(* Logix 5000 AddOnInstructionDefinition export MPLS_Yaskawa; software revision 17.00 *)

TYPE Yaskawa_PLS_Switch :   // Structure of parameters needed for PLS switch operation using MPLS_Yaskawa v2.4.0
STRUCT
   FlagNumber : INT;   // Assigns a Flag number to the PLS output channel. Must be a physical output Flag 73-80, 88-90.
   OnPosition : REAL;   // If OnPosition < OffPosition output is ON between them. If OnPosition > OffPosition output is OFF between them and ON everywhere else.
   OffPosition : REAL;
   OnCompensation : INT;   // [msec]. Negative number turns output on SOONER, positive number turns output on LATER.
   OffCompensation : INT;   // [msec]
END_STRUCT
END_TYPE

TYPE Yaskawa_EIP_Servo :   // Yaskawa SigmaLogic Axis Structure v2.4.0
STRUCT
   O : Yaskawa_OUT_to_Servo;
   I : Yaskawa_IN_from_Servo;
   AOI_SB : Yaskawa_AOI_Status_Bits;
END_STRUCT
END_TYPE

TYPE Yaskawa_OUT_to_Servo :   // Structure of data sent out to the Yaskawa SigmaLogic controller v2.4.0
STRUCT
   b00_ServoOn : BOOL;   // Servo On
   b01_Stop : BOOL;   // Stops All Current Motion in Progress
   b02_Home : BOOL;   // Start Homing Process
   b03_MoveStart1 : BOOL;   // Start Current Motion
   b06_SuperImpose : BOOL;
   b07_ServoAlarmReset : BOOL;   // Servo Alarm Reset
   b08_ControllerAlarmReset : BOOL;   // SigmaLogic Alarm Reset
   b09_MoveStart2 : BOOL;   // Start Second Motion (Blended Move)
   b10_MoveAbort : BOOL;   // Abort Current Move
   b11_MovePause : BOOL;   // Pause Current Move
   b12_SeqPause : BOOL;   // Indexing Sequence Pause
   b13_SeqResume : BOOL;   // Indexing Sequence Resume
   b14_SeqCancel : BOOL;   // Indexing Sequence Cancel
   b15_AbsEncoderReset : BOOL;   // Absolute Encoder Reset
   b16_SeqStart : BOOL;   // Start Indexing Sequence
   b17_SeqEditSpeed : BOOL;   // Enter Edit Speed
   b18_SeqEditDistance : BOOL;   // Enter Distance Edit
   b19_PLSEnable : BOOL;   // Enable PLS execution
   b20_PLSActivateOutput1 : BOOL;   // Activate PLS output1 switch logic
   b21_PLSActivateOutput2 : BOOL;   // Activate PLS output2 switch logic
   b22_PLSActivateOutput3 : BOOL;   // Activate PLS output3 switch logic
   b23_PLSActivateOutput4 : BOOL;   // Activate PLS output4 switch logic
   b24_SetClock : BOOL;   // Set the remote controller clock with data provided by the PLC
   RebootController : BOOL;
   UseExternalEncoder : BOOL;   // Use External Encoder when executing MAHSP_Yaskawa
   b32_HeatbeatAnswer : BOOL;   // Heartbeat Answer
   BrakeBypassRequest : BOOL;
   SetFwdTorqueLimit : BOOL;
   SetRevTorqueLimit : BOOL;
   TorqueLimit : DINT;
   TorqueRamp : DINT;
   HomeMethod : INT;
   HomeSpeed : DINT;
   HomeAccDec : DINT;   // Home Move Acceleration/Deceleration Rate
   HomeBackOffDistance : DINT;
   HomeCreepSpeed : DINT;
   HomeCreepDistanceLimit : DINT;
   HomeCreepTimeLimit : DINT;
   HomeOffsetDistance : DINT;
   HomeOffsetSpeed : DINT;
   HomePostion : DINT;
   HomeTorque : DINT;
   HomeInputNo : DINT;
   HomeApproachTimeLimit : DINT;
   HomeApproachDistLimit : DINT;
   HomeDirection : INT;
   HomeSwitchMode : INT;
   MoveType : INT;
   MoveDirection : INT;
   MoveAccel1 : DINT;
   MoveAccel2 : DINT;
   MoveDecel1 : DINT;
   MoveDecel2 : DINT;
   MoveSpeed1 : DINT;
   MoveSpeed2 : DINT;
   MoveDistance1 : DINT;
   MoveDistance2 : DINT;
   MovePosition1 : DINT;
   MovePosition2 : DINT;
   RegistrationDistance : DINT;
   GearNumerator : DINT;
   GearDenominator : DINT;
   SuperImposeDistance : DINT;
   Resolution : INT;
   RegistrationDirection : INT;
   TuningLevel : INT;
   SequenceStep : INT;   // Staring Sequence Step Number
   SequenceEditStep : INT;   // Sequence Step Number to Edit
   FlagCommandBits1 : DINT;   // Flag Commands. 1..64 are General Flags, Bits 0..31 correspond to Flag 1..32
   FlagCommandBits2 : DINT;   // Flag Commands cont. 1..64 are General Flags, Bits 0..31 correspond to Flag 33..64
   DigitalOutCommandBits : DINT;   // Digital Output commands. Bits 0-7 correspond to CN13 Digital Outputs 0-7, used as Flag 73-80. Bits 8-10 correspond to CN1 Digital Outputs 0-2 used as Flag 88-90"
   SequenceEditSpeed : DINT;
   SequenceEditDistance : DINT;
   FeedRateOverride : INT;
   HSI_Enable : BOOL;
   HSI_MoveMode : BOOL;   // 0=Relative; 1=Moves per Cycle
   HSI_CalcMethod : BOOL;   // 0=Accel/Decel; 1=Time
   HSI_MoveDirection : BOOL;   // 0 = Negative; 1 = Positive
   HSI_TriggerFlag : INT;
   HSI_MovingFlag : INT;
   HSI_DwellingFlag : INT;
   HSI_DoneFlag : INT;
   HSI_MoveType : INT;   // 0=Single; 1=Repeat; 2=Repeat "x" times
   HSI_RepeatNumber : INT;
   HSI_Distance : DINT;
   HSI_Speed : DINT;
   HSI_Accel : DINT;
   HSI_MoveTime : DINT;
   HSI_DwellTime : DINT;
   PLS_OutputFlag1 : INT;
   PLS_OutputFlag2 : INT;
   PLS_OutputFlag3 : INT;
   PLS_OutputFlag4 : INT;
   PLS_OnPosition1 : DINT;
   PLS_OffPosition1 : DINT;
   PLS_OnPosition2 : DINT;
   PLS_OffPosition2 : DINT;
   PLS_OnPosition3 : DINT;
   PLS_OffPosition3 : DINT;
   PLS_OnPosition4 : DINT;
   PLS_OffPosition4 : DINT;
   PLS_OnCompensation1 : INT;
   PLS_OffCompensation1 : INT;
   PLS_OnCompensation2 : INT;
   PLS_OffCompensation2 : INT;
   PLS_OnCompensation3 : INT;
   PLS_OffCompensation3 : INT;
   PLS_OnCompensation4 : INT;
   PLS_OffCompensation4 : INT;
   RTC_Year : INT;
   RTC_Month : INT;
   RTC_Day : INT;
   RTC_Hour : INT;
   RTC_Min : INT;
   RTC_Sec : INT;
   StopDecel : DINT;
   AnalogOutput : INT;   // CN13, AO_01 [mV]
END_STRUCT
END_TYPE

TYPE Yaskawa_AOI_Status_Bits :   // Internal bits used to interlock Yaskawa AOI execution. v2.4.0
STRUCT
   MAM : BOOL;   // Move AOI Active
   MAJ : BOOL;   // Jog AOI Active
   MAB : BOOL;   // Blending AOI Active
   MAG : BOOL;   // Gearing AOI Active
   MAHSP : BOOL;   // Home SetPoint AOI Active
   MAH : BOOL;   // Homing AOI Active
   MSQE : BOOL;   // Sequence Edit AOI Active
   MSQR : BOOL;   // Sequence Run AOI Active
   MHSI : BOOL;   // High Speed Index AOI Active
   MSO : BOOL;   // Servo On
   MSF : BOOL;   // Servo Off
   MAFR : BOOL;   // Fault Reset
   MAS : BOOL;   // Servo Abort
   MTRQ : BOOL;   // Torque Mode Active
   MPLS : BOOL;   // PLS Active
   MCLK : BOOL;   // SetClock Active
   MSTL : BOOL;   // Set Torque Limit Active
   AOI_Permissive : BOOL;   // Permissive to Execute an AOI
END_STRUCT
END_TYPE

TYPE Yaskawa_IN_from_Servo :   // Structure of data coming from the Yaskawa SigmaLogic controller. v2.4.0
STRUCT
   AlarmText : STRING;   // ServoPack Alarm Code plus Text Description
   b00_Heartbeat : BOOL;
   b01_Alarm : BOOL;   // ServoPack Alarm
   b02_Warning : BOOL;   // ServoPack Warning
   b03_Ready : BOOL;   // ServoPack Ready
   b04_Enabled : BOOL;   // ServoPack Enabled ("Servo On")
   b05_StopComplete : BOOL;
   b06_HomeComplete : BOOL;
   b07_HomeBusy : BOOL;
   b08_HomeActive : BOOL;
   b09_HomeAborted : BOOL;
   b10_HomeError : BOOL;
   b11_MoveAbsComplete : BOOL;
   b12_MoveAbsBusy : BOOL;
   b13_MoveAbsActive : BOOL;
   b14_MoveAbsAborted : BOOL;
   b15_MoveAbsError : BOOL;
   b16_MoveRelComplete : BOOL;
   b17_MoveRelBusy : BOOL;
   b18_MoveRelActive : BOOL;
   b19_MoveRelAborted : BOOL;
   b20_MoveRelError : BOOL;
   b21_JogAtSpeed : BOOL;
   b22_JogBusy : BOOL;
   b23_JogActive : BOOL;
   b24_JogAborted : BOOL;
   b25_JogError : BOOL;
   b26_GearInSync : BOOL;
   b27_GearBusy : BOOL;
   b28_GearActive : BOOL;
   b29_GearAborted : BOOL;
   b30_GearError : BOOL;
   b32_MoveSuperComplete : BOOL;
   b33_MoveSuperBusy : BOOL;
   b34_MoveSuperActive : BOOL;
   b35_MoveSuperAborted : BOOL;
   b36_MoveSuperError : BOOL;
   b37_PowerCycleRequired : BOOL;
   b38_MoveBlend1Complete : BOOL;
   b39_MoveBlend1Busy : BOOL;
   b40_MoveBlend1Active : BOOL;
   b41_MoveBlend1Abort : BOOL;
   b42_MoveBlend1Error : BOOL;
   b43_MoveBlend2Complete : BOOL;
   b44_MoveBlend2Busy : BOOL;
   b45_MoveBlend2Active : BOOL;
   b46_MoveBlend2Abort : BOOL;
   b47_MoveBlend2Error : BOOL;
   b48_RegComplete : BOOL;
   b49_RegBusy : BOOL;
   b50_RegActive : BOOL;
   b51_RegAborted : BOOL;
   b52_RegError : BOOL;
   b53_ResetAbsEncoderActive : BOOL;
   b54_ResetAbsEncoderBusy : BOOL;
   b55_ResetAbsEncoderDone : BOOL;
   b56_ResetAbsEncoderError : BOOL;
   b57_SeqRunning : BOOL;
   b58_RegSensorNotReached : BOOL;
   b59_SeqEditError : BOOL;
   b60_SeqEditDone : BOOL;
   b61_TorqueAtTorque : BOOL;
   b62_TorqueBusy : BOOL;
   b63_TorqueActive : BOOL;
   b64_TorqueAborted : BOOL;
   b65_TorqueError : BOOL;
   b66_ControllerAlarm : BOOL;
   b67_ApplicationError : BOOL;
   b68_AxisAtStandStill : BOOL;
   b69_TestModeActive : BOOL;
   b70_ServoParamsOK : BOOL;
   b71_SetFwdTorqueLimitDone : BOOL;
   b72_SetRevTorqueLimitDone : BOOL;
   Position : DINT;
   Speed : DINT;
   Torque : DINT;
   HomeErrorID : INT;
   MoveAbsErrorID : INT;
   MoveRelErrorID : INT;
   JogErrorID : INT;
   GearErrorID : INT;
   MoveSuperErrorID : INT;
   ServoAlarmID : INT;
   ServoWarningID : INT;
   ControllerAlarmID : DINT;
   AxisGenAlarmID : DINT;
   MoveBlend1ErrorID : INT;
   MoveBlend2ErrorID : INT;
   ResetAbsEncoderErrorID : INT;
   FunctionBlockErrorID : INT;
   TorqueErrorID : INT;
   RegErrorID : INT;
   SeqCurrentStep : INT;
   FlagStatusBit1 : DINT;   // Flag Status. 1..64 are General Flags, Bits 0..31 correspond to Flag 1..32
   FlagStatusBit2 : DINT;   // Flag Status cont. 1..64 are General Flags, Bits 0..31 correspond to Flag 33..64
   IOStatusBits : DINT;   // Digital IO Status. Bits 0-7, CN13 Inputs 0-7, Used as Flag 65-72. Bits 8-15, CN13 Outputs 0-7, Used as Flag 73-80. Bits 16-22, CN1 Inputs 0-6, Used as Flag 81-87. Bits 23-25, CN1 Outputs 0-4, Used as Flag 88-92.
   HSI_Moving : BOOL;
   HSI_Dwelling : BOOL;
   HSI_Done : BOOL;
   HSI_Busy : BOOL;
   HSI_Error : BOOL;
   HSI_ErrorCode : INT;
   PLS_Running : BOOL;
   PLS_SwitchStatus1 : BOOL;
   PLS_SwitchStatus2 : BOOL;
   PLS_SwitchStatus3 : BOOL;
   PLS_SwitchStatus4 : BOOL;
   PLS_Busy : BOOL;
   PLS_Error : BOOL;
   PLS_ErrorCode : INT;
   SetClock_Done : BOOL;
   SetClock_Busy : BOOL;
   SetClock_Error : BOOL;
   SetClock_ErrorID : INT;
   SoftwareVersion : DINT;
   FirmwareVersion : DINT;
   CommandedPos : DINT;
   CommandedPosNonCyc : DINT;
   CommandedSpeed : DINT;
   Clock_Year : INT;
   Clock_Month : INT;
   Clock_Day : INT;
   Clock_Hour : INT;
   Clock_Minute : INT;
   Clock_Second : INT;
   AnalogInput : REAL;   // CN13, AI_01 [v]
   BrakeBypassActive : BOOL;
   ForwardTorqueLimit : DINT;
   ReverseTorqueLimit : DINT;
END_STRUCT
END_TYPE

ADD_ON_INSTRUCTION MPLS_Yaskawa   (* revision 2.4 0, vendor Yaskawa America, Inc., ExecuteEnableInFalse *)
// Motion Programmable Limit Switch
// Revision note:
// 2.4.0: No functional change
// 2.3.1: No functional change
// 2.3.0: No functional change
// 2.0.0: Improved output operation and error code reporting. Improved interlocking with embedded code.
// 1.2.0: No functional change.
// Initial Release 9/10/2014
// Help:
// This AOI transfers settings to the remote axis node for high-response of local outputs in relation to servo position. This block can run simultaneously with other motion function blocks. Up to four local digital outputs can be configured as a PLS output. Each has a single switch for OnPosition and OffPosition in relation to the servo axis position. Automatic Speed Compensation is supported independently for the OnPosition and for the OffPosition. Output Time Duration limiting is NOT supported at this time. However, the main PLC can easily monitor the switch output signals and deactivate the switch from the application code if a certain time limit is exceeded.
// SwitchData is a structure consisting of:
// - FlagNumber [INT]
// - OnPosition [REAL]
// - OffPosition [REAL]
// - OnCompensation [INT]
// - OffCompensation [INT]
VAR_IN_OUT
   Axis : Yaskawa_EIP_Servo; {required}
END_VAR
VAR_OUTPUT
   EN : BOOL; {visible}   // AOI is Active
   DN : BOOL; {visible}   // PLS_Busy
   IP : BOOL; {visible}   // PLS_Running
   ER : BOOL; {visible}   // PLS_Error
END_VAR
VAR_IN_OUT
   Switch1Data : Yaskawa_PLS_Switch; {required}
   Switch2Data : Yaskawa_PLS_Switch; {required}
   Switch3Data : Yaskawa_PLS_Switch; {required}
   Switch4Data : Yaskawa_PLS_Switch; {required}
END_VAR
VAR_INPUT
   ActivateSwitch1 : BOOL; {required}
   ActivateSwitch2 : BOOL; {required}
   ActivateSwitch3 : BOOL; {required}
   ActivateSwitch4 : BOOL; {required}
END_VAR
VAR_OUTPUT
   S1 : BOOL; {visible}   // Switch1 Status
   S2 : BOOL; {visible}   // Switch2 Status
   S3 : BOOL; {visible}   // Switch3 Status
   S4 : BOOL; {visible}   // Switch4 Status
   FLT_RDY : BOOL; {visible}   // The Servo is Not Ready
   FLT_BSY : BOOL;   // There is another AOI Active for this Axis
   ErrorCode : DINT; {visible}   // Fault code for PLS function
END_VAR
VAR
   AOI_ON_LOCAL : BOOL;
   ScaleFactor : DINT;
END_VAR

ROUTINE EnableInFalse   (* ladder *)
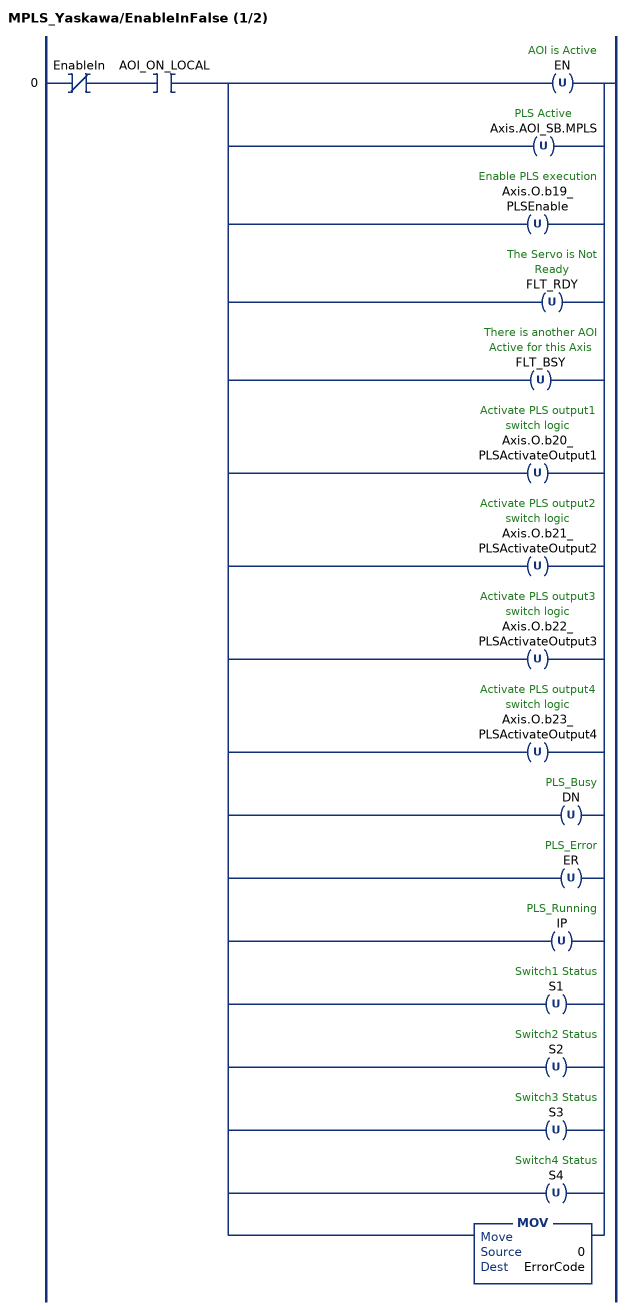
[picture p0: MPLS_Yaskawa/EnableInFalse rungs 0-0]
   0: XIO(EnableIn)XIC(AOI_ON_LOCAL)[OTU(EN) ,OTU(Axis.AOI_SB.MPLS) ,OTU(Axis.O.b19_PLSEnable) ,OTU(FLT_RDY) ,OTU(FLT_BSY) ,OTU(Axis.O.b20_PLSActivateOutput1) ,OTU(Axis.O.b21_PLSActivateOutput2) ,OTU(Axis.O.b22_PLSActivateOutput3) ,OTU(Axis.O.b23_PLSActivateOutput4) ,OTU(DN) ,OTU(ER) ,OTU(IP) ,OTU(S1) ,OTU(S2) ,OTU(S3) ,OTU(S4) ,MOV(0,ErrorCode) ];
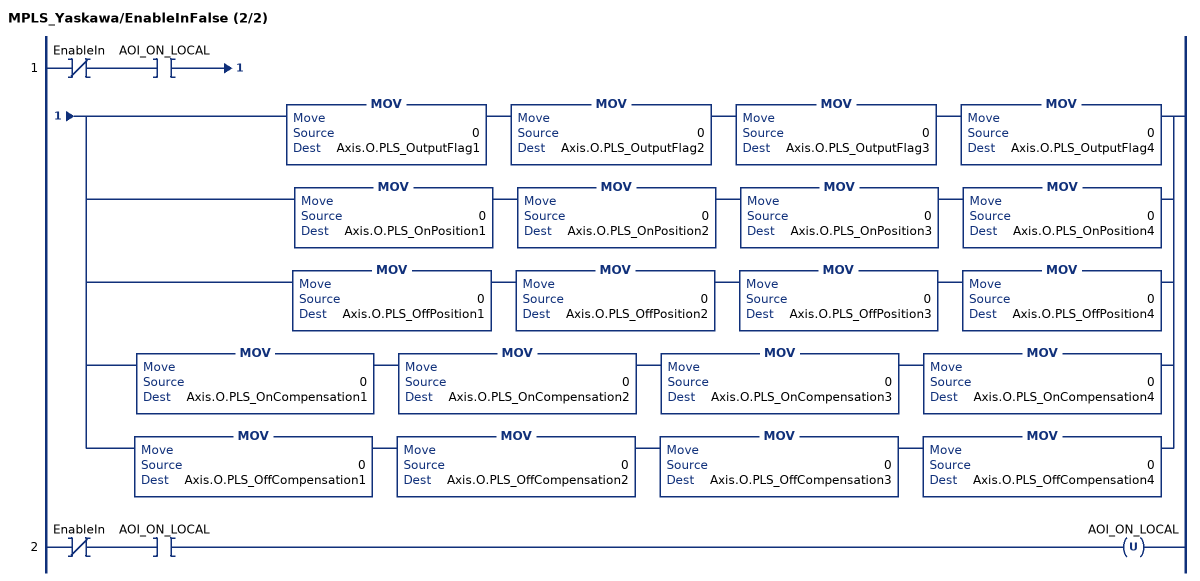
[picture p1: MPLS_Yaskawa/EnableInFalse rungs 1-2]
   1: XIO(EnableIn)XIC(AOI_ON_LOCAL)[MOV(0,Axis.O.PLS_OutputFlag1) MOV(0,Axis.O.PLS_OutputFlag2) MOV(0,Axis.O.PLS_OutputFlag3) MOV(0,Axis.O.PLS_OutputFlag4) ,MOV(0,Axis.O.PLS_OnPosition1) MOV(0,Axis.O.PLS_OnPosition2) MOV(0,Axis.O.PLS_OnPosition3) MOV(0,Axis.O.PLS_OnPosition4) ,MOV(0,Axis.O.PLS_OffPosition1) MOV(0,Axis.O.PLS_OffPosition2) MOV(0,Axis.O.PLS_OffPosition3) MOV(0,Axis.O.PLS_OffPosition4) ,MOV(0,Axis.O.PLS_OnCompensation1) MOV(0,Axis.O.PLS_OnCompensation2) MOV(0,Axis.O.PLS_OnCompensation3) MOV(0,Axis.O.PLS_OnCompensation4) ,MOV(0,Axis.O.PLS_OffCompensation1) MOV(0,Axis.O.PLS_OffCompensation2) MOV(0,Axis.O.PLS_OffCompensation3) MOV(0,Axis.O.PLS_OffCompensation4) ];
   2: XIO(EnableIn)XIC(AOI_ON_LOCAL)OTU(AOI_ON_LOCAL);
END_ROUTINE

ROUTINE Logic   (* ladder *)
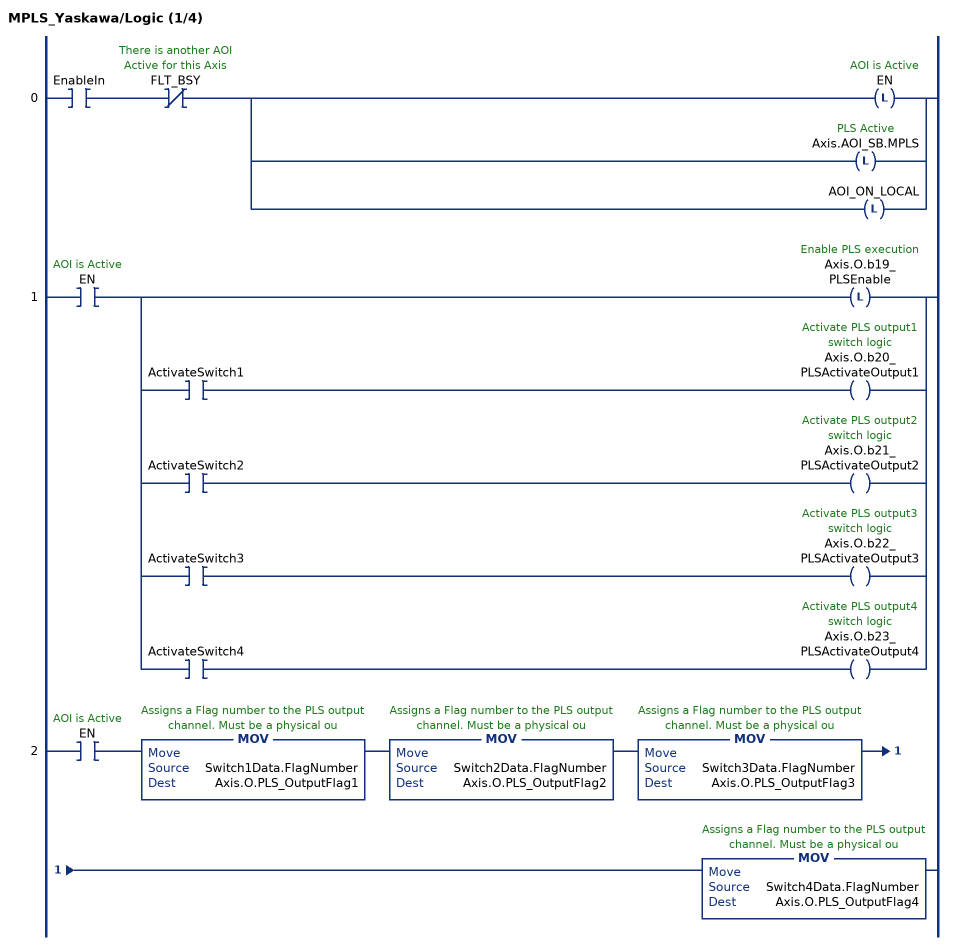
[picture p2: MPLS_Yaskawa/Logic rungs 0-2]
   0: XIC(EnableIn)XIO(FLT_BSY)[OTL(EN) ,OTL(Axis.AOI_SB.MPLS) ,OTL(AOI_ON_LOCAL) ];
   1: XIC(EN)[OTL(Axis.O.b19_PLSEnable) ,XIC(ActivateSwitch1) OTE(Axis.O.b20_PLSActivateOutput1) ,XIC(ActivateSwitch2) OTE(Axis.O.b21_PLSActivateOutput2) ,XIC(ActivateSwitch3) OTE(Axis.O.b22_PLSActivateOutput3) ,XIC(ActivateSwitch4) OTE(Axis.O.b23_PLSActivateOutput4) ];
   2: XIC(EN)MOV(Switch1Data.FlagNumber,Axis.O.PLS_OutputFlag1)MOV(Switch2Data.FlagNumber,Axis.O.PLS_OutputFlag2)MOV(Switch3Data.FlagNumber,Axis.O.PLS_OutputFlag3)MOV(Switch4Data.FlagNumber,Axis.O.PLS_OutputFlag4);
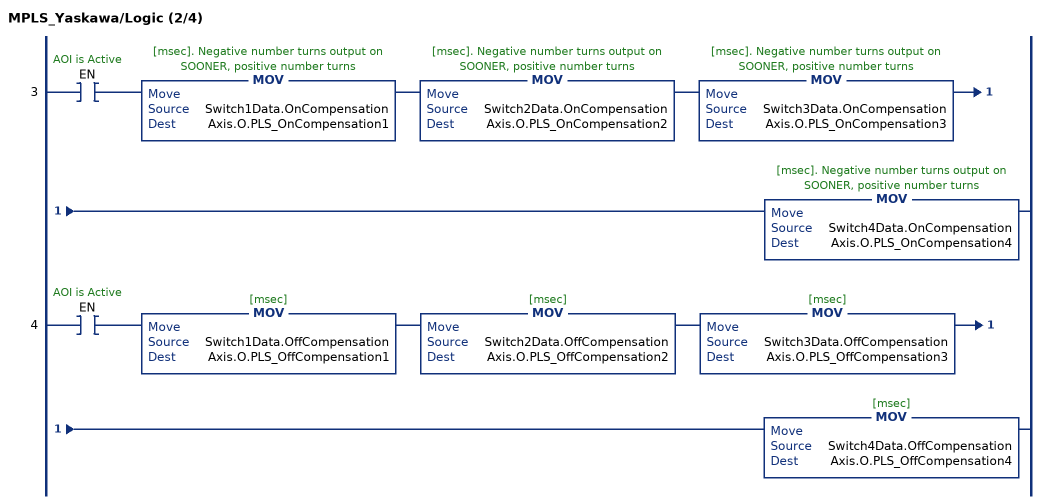
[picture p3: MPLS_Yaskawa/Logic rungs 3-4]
   3: XIC(EN)MOV(Switch1Data.OnCompensation,Axis.O.PLS_OnCompensation1)MOV(Switch2Data.OnCompensation,Axis.O.PLS_OnCompensation2)MOV(Switch3Data.OnCompensation,Axis.O.PLS_OnCompensation3)MOV(Switch4Data.OnCompensation,Axis.O.PLS_OnCompensation4);
   4: XIC(EN)MOV(Switch1Data.OffCompensation,Axis.O.PLS_OffCompensation1)MOV(Switch2Data.OffCompensation,Axis.O.PLS_OffCompensation2)MOV(Switch3Data.OffCompensation,Axis.O.PLS_OffCompensation3)MOV(Switch4Data.OffCompensation,Axis.O.PLS_OffCompensation4);
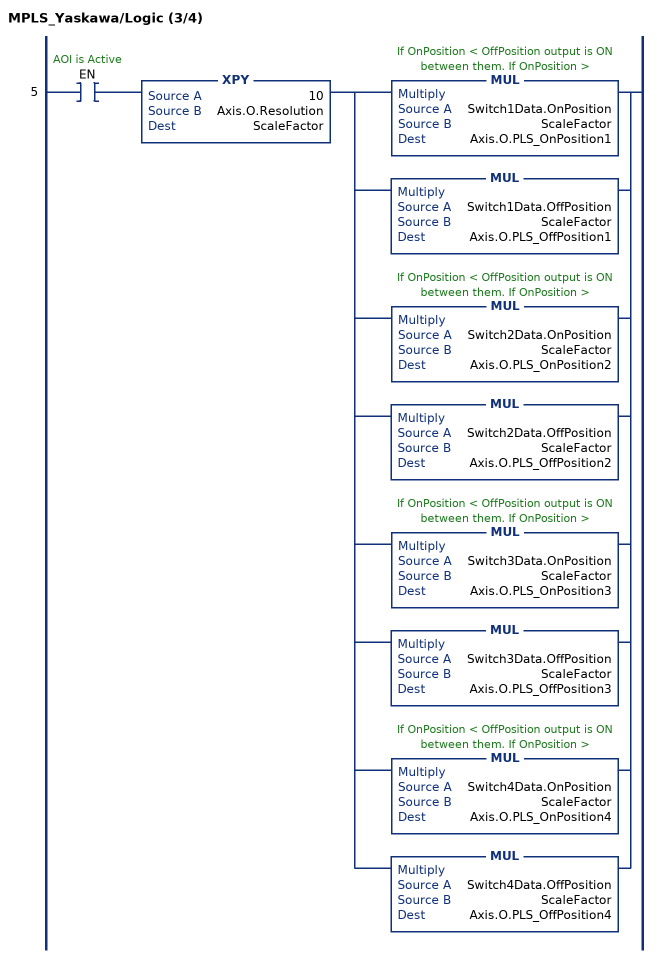
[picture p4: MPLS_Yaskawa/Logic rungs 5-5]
   5: XIC(EN)XPY(10,Axis.O.Resolution,ScaleFactor)[MUL(Switch1Data.OnPosition,ScaleFactor,Axis.O.PLS_OnPosition1) ,MUL(Switch1Data.OffPosition,ScaleFactor,Axis.O.PLS_OffPosition1) ,MUL(Switch2Data.OnPosition,ScaleFactor,Axis.O.PLS_OnPosition2) ,MUL(Switch2Data.OffPosition,ScaleFactor,Axis.O.PLS_OffPosition2) ,MUL(Switch3Data.OnPosition,ScaleFactor,Axis.O.PLS_OnPosition3) ,MUL(Switch3Data.OffPosition,ScaleFactor,Axis.O.PLS_OffPosition3) ,MUL(Switch4Data.OnPosition,ScaleFactor,Axis.O.PLS_OnPosition4) ,MUL(Switch4Data.OffPosition,ScaleFactor,Axis.O.PLS_OffPosition4) ];
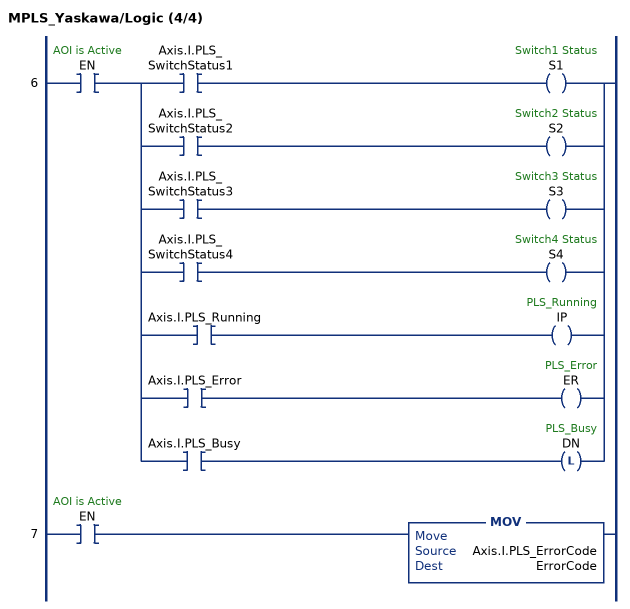
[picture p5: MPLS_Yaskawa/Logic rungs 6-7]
   6: XIC(EN)[XIC(Axis.I.PLS_SwitchStatus1) OTE(S1) ,XIC(Axis.I.PLS_SwitchStatus2) OTE(S2) ,XIC(Axis.I.PLS_SwitchStatus3) OTE(S3) ,XIC(Axis.I.PLS_SwitchStatus4) OTE(S4) ,XIC(Axis.I.PLS_Running) OTE(IP) ,XIC(Axis.I.PLS_Error) OTE(ER) ,XIC(Axis.I.PLS_Busy) OTL(DN) ];
   7: XIC(EN)MOV(Axis.I.PLS_ErrorCode,ErrorCode);
END_ROUTINE
END_ADD_ON_INSTRUCTION
